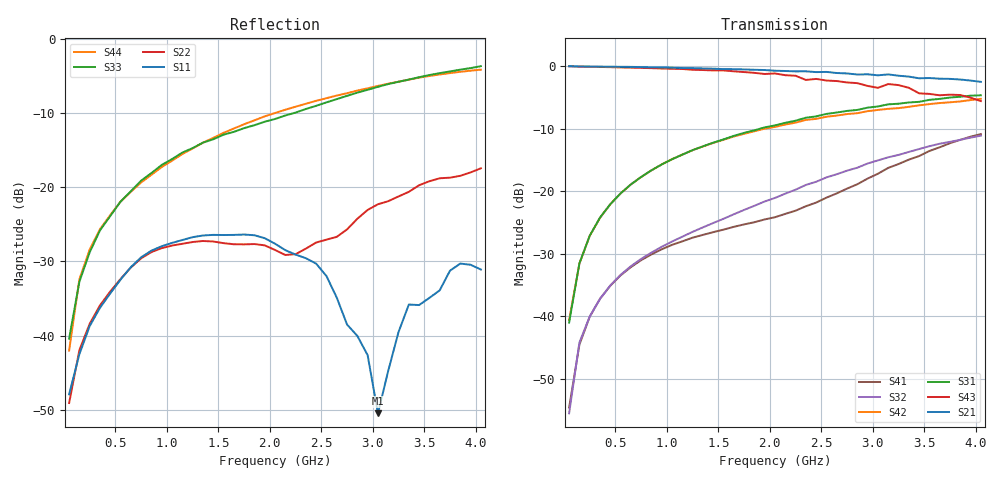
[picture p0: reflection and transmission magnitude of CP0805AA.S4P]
! Network Analyzer HP8720D.07.14 Serial No. US38111185
! 28 Apr 1999  02:06:29
! Frequency 	S11		S21		S31		S41		S12		S22		S23		S24		S13		S23		S33		S34		S14		S24		S34		S44
# HZ  S  DB R 50
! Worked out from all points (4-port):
!   41 points, 50 MHz to 4.05 GHz, reference 50 ohm
!   strongest paths, dB at 50 MHz, 1.05 GHz, 2.05 GHz, 3.05 GHz, 4.05 GHz:
!     S21: 0.0, -0.2, -0.7, -1.4, -2.5
!     S43: 0.0, -0.4, -1.1, -3.4, -5.6
!     S31: -41.0, -14.9, -9.5, -6.4, -4.6
!     S42: -40.6, -14.9, -9.7, -7.0, -5.2
!     S32: -55.5, -28.0, -21.1, -15.1, -11.1
!     S41: -54.6, -28.6, -24.2, -17.2, -10.8
!   lowest |S11| = -50.5 dB at 3.05 GHz (marker M1), VSWR 1.01, Z = 50.2 + j0.235 ohm
!   |S11| at or under -10 dB: start of sweep to end of sweep
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5e7  -47.92 -30.7  -0.01 -1.0  -40.13 95.7  -52.70 96.8
     0.03 -1.0  -49.09 -11.2  -53.45 99.5  -40.87 89.5
     -41.02 89.6  -55.54 76.8  -40.42 61.5  -0.02 -1.6
     -54.62 97.1  -40.60 89.2  0.00 -1.6  -42.04 61.7
4.5e8  -34.32 -110.2  -0.07 -9.6  -22.05 78.6  -35.12 81.5
       -0.07 -9.7  -34.07 -95.6  -35.09 84.4  -22.07 77.8
       -22.06 78.4  -35.09 84.3  -23.90 60.4  -0.13 -14.1
       -35.11 81.5  -22.08 77.7  -0.13 -14.3  -23.77 57.6
1.75e9  -26.40 153.0  -0.50 -36.9  -10.59 46.7  -25.22 71.9
        -0.50 -36.2  -27.72 -171.2  -22.90 79.8  -10.70 43.1
        -10.65 47.8  -22.98 80.7  -12.06 -3.6  -0.96 -55.2
        -25.30 73.0  -10.80 44.1  -0.92 -56.7  -11.54 -3.2
2.55e9  -32.00 105.1  -1.00 -52.9  -7.82 25.4  -21.06 80.3
        -0.89 -52.7  -27.08 92.4  -17.99 70.4  -8.11 20.8
        -7.61 28.0  -17.77 73.0  -8.59 -57.3  -2.05 -83.1
        -21.01 83.4  -8.06 23.4  -2.27 -79.7  -8.03 -34.7
3.05e9  -50.48 51.6  -1.34 -62.7  -6.70 12.7  -17.17 78.7
        -1.44 -62.4  -22.32 41.4  -15.44 61.0  -7.06 7.9
        -6.42 16.6  -15.05 64.7  -6.50 -88.0  -2.84 -101.0
        -17.19 83.3  -6.98 12.2  -3.44 -99.3  -6.37 -59.8
3.35e9  -35.83 -126.2  -1.56 -68.7  -5.54 7.6  -14.59 76.6
        -1.64 -69.1  -20.65 20.7  -13.52 55.9  -6.23 4.2
        -5.78 8.8  -13.70 57.7  -5.52 -105.6  -3.06 -108.6
        -14.93 77.1  -6.48 5.2  -3.43 -110.9  -5.54 -76.7
4.05e9  -31.11 145.3  -2.16 -81.7  -5.16 -14.1  -10.92 50.0
        -2.48 -82.1  -17.48 -4.0  -11.90 33.7  -5.57 -17.3
        -4.63 -8.0  -11.10 39.8  -3.71 -143.7  -4.88 -142.6
        -10.85 57.0  -5.20 -10.2  -5.56 -140.3  -4.18 -117.8
